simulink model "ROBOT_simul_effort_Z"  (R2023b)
settings: Solver=VariableStepAuto  StartTime=0.0  StopTime=5  RelTol=1e-3
undefined symbols (not defined in the file): deg, kg, m, manette1_Defaut_sldprt, manette2_Defaut_sldprt, mm, N, rad, s, STL, X, Y, Z
libraries: sm_lib x463, fl_lib x45, nesl_utility x27, simulink x2
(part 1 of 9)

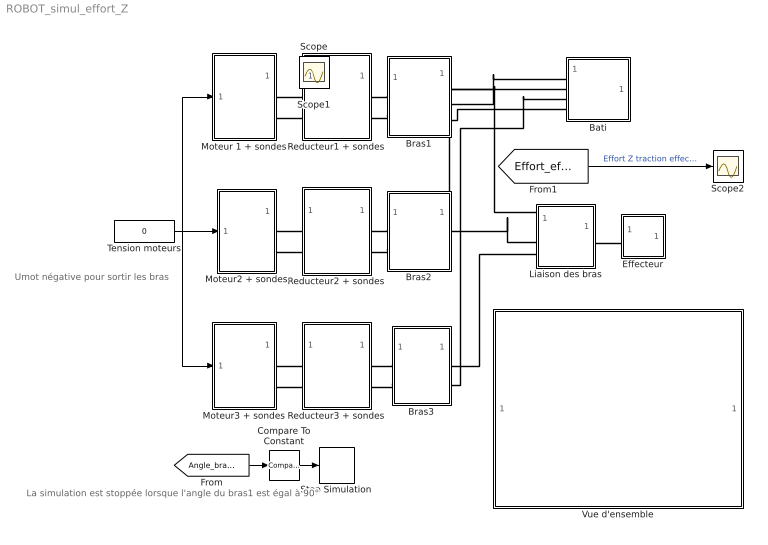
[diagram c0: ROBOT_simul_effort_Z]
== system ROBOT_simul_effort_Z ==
  note: La simulation est stoppée lorsque l'angle du bras1 est égal à 90°
  note: Umot négative pour sortir les bras
  Bati : Subsystem
  Bras1 : Subsystem
  Bras2 : Subsystem
  Bras3 : Subsystem
  Compare To Constant : simulink/Logic and Bit Operations/Compare To Constant  relop=>=  const=85  OutDataTypeStr=boolean
  Effecteur : Subsystem
  Liaison des bras : Subsystem
  Moteur 1 + sondes : Subsystem
  Moteur2 + sondes : Subsystem
  Moteur3 + sondes : Subsystem
  Reducteur1 + sondes : Subsystem
  Reducteur2 + sondes : Subsystem
  Reducteur3 + sondes : Subsystem
  Scope2 : Scope
  Stop Simulation : Stop
  Tension moteurs : Constant  Value=0
  Vue d'ensemble : Subsystem
  Scope : Scope
  Scope1 : Scope
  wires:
  [Angle_bras1] -> Compare To Constant/1
  Compare To Constant/1 -> Stop Simulation/1
  Tension moteurs/1 -> Moteur2 + sondes/1(In1), Moteur 1 + sondes/1(In1), Moteur3 + sondes/1(In1)
  [Effort_effecteur] -> Scope2/1  "Effort Z traction effecteur (N)"
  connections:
  Bras3/RConn2 -- Bati/LConn3
  Bras1/LConn2 -- Reducteur1 + sondes/RConn2
  Bras2/RConn2 -- Bati/LConn2
  Moteur3 + sondes/RConn2 -- Reducteur3 + sondes/LConn2
  Bras1/RConn2 -- Bati/LConn1
  Bras1/RConn3 -- Bati/LConn4
  Liaison des bras/LConn1 -- Bras1/RConn1
  Bras3/LConn1 -- Reducteur3 + sondes/RConn1
  Moteur 1 + sondes/RConn1 -- Reducteur1 + sondes/LConn1
  Liaison des bras/LConn3 -- Bras3/RConn1
  Liaison des bras/RConn1 -- Effecteur/LConn1
  Liaison des bras/LConn2 -- Bras2/RConn1
  Moteur2 + sondes/RConn1 -- Reducteur2 + sondes/LConn1
  Bras1/LConn1 -- Reducteur1 + sondes/RConn1
  Bras3/LConn2 -- Reducteur3 + sondes/RConn2
  Moteur2 + sondes/RConn2 -- Reducteur2 + sondes/LConn2
  Bras2/LConn2 -- Reducteur2 + sondes/RConn2
  Moteur 1 + sondes/RConn2 -- Reducteur1 + sondes/LConn2
  Bras2/LConn1 -- Reducteur2 + sondes/RConn1
  Moteur3 + sondes/RConn1 -- Reducteur3 + sondes/LConn1

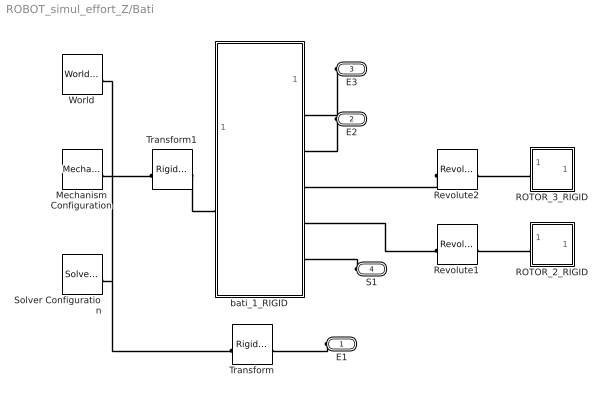
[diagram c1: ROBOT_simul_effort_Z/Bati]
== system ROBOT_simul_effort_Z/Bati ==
  Mechanism Configuration : sm_lib/Utilities/Mechanism Configuration  UniformGravity=Constant  GravityVector=[0 -9.81 0]  GravityVectorUnits=m/s^2  LinearizationDelta=0.001  JointModeTransitionNonlinearIterations=2
  ROTOR_2_RIGID : Subsystem
  ROTOR_3_RIGID : Subsystem
  Revolute1 : sm_lib/Joints/Revolute Joint  JointMode=Normal  SenseConstraintForce=off  SenseConstraintForceX=off  SenseConstraintForceY=off  SenseConstraintForceZ=off  SenseConstraintTorque=off  SenseConstraintTorqueX=off  SenseConstraintTorqueY=off  SenseConstraintTorqueZ=off  SenseTotalForce=off  SenseTotalForceX=off  SenseTotalForceY=off  SenseTotalForceZ=off  SenseTotalTorque=off  SenseTotalTorqueX=off  SenseTotalTorqueY=off  SenseTotalTorqueZ=off  CompositeWrenchDir=FollowerOnBase  CompositeWrenchFrame=BaseFrame  EquilibriumPosition=0  EquilibriumPositionUnits=rad  SpringStiffness=0  SpringStiffnessUnits=m*N/rad  DampingCoefficient=0  DampingCoefficientUnits=m*s*N/rad  TorqueActuationMode=NoTorque  MotionActuationMode=ComputedMotion  SensePosition=off  SenseVelocity=off  SenseAcceleration=off  SenseTorqueForce=off  SenseLowerLimitTorqueForce=off  SenseUpperLimitTorqueForce=off  LowerLimitSpecify=off  LowerLimitBound=-90  LowerLimitBoundUnits=deg  LowerLimitStiffness=1e4  LowerLimitStiffnessUnits=N*m/deg  LowerLimitDamping=10  LowerLimitDampingUnits=N*m/(deg/s)  LowerLimitTransitionRegionWidth=0.1  LowerLimitTransitionRegionWidthUnits=deg  UpperLimitSpecify=off  UpperLimitBound=90  UpperLimitBoundUnits=deg  UpperLimitStiffness=1e4  UpperLimitStiffnessUnits=N*m/deg  UpperLimitDamping=10  UpperLimitDampingUnits=N*m/(deg/s)  UpperLimitTransitionRegionWidth=0.1  UpperLimitTransitionRegionWidthUnits=deg  PositionTargetSpecify=on  PositionTargetPriority=Low  PositionTargetValue=-26.406351854743253  PositionTargetValueUnits=deg  VelocityTargetSpecify=off  VelocityTargetPriority=High  VelocityTargetValue=0  VelocityTargetValueUnits=deg/s
  Revolute2 : sm_lib/Joints/Revolute Joint  JointMode=Normal  SenseConstraintForce=off  SenseConstraintForceX=off  SenseConstraintForceY=off  SenseConstraintForceZ=off  SenseConstraintTorque=off  SenseConstraintTorqueX=off  SenseConstraintTorqueY=off  SenseConstraintTorqueZ=off  SenseTotalForce=off  SenseTotalForceX=off  SenseTotalForceY=off  SenseTotalForceZ=off  SenseTotalTorque=off  SenseTotalTorqueX=off  SenseTotalTorqueY=off  SenseTotalTorqueZ=off  CompositeWrenchDir=FollowerOnBase  CompositeWrenchFrame=BaseFrame  EquilibriumPosition=0  EquilibriumPositionUnits=rad  SpringStiffness=0  SpringStiffnessUnits=m*N/rad  DampingCoefficient=0  DampingCoefficientUnits=m*s*N/rad  TorqueActuationMode=NoTorque  MotionActuationMode=ComputedMotion  SensePosition=off  SenseVelocity=off  SenseAcceleration=off  SenseTorqueForce=off  SenseLowerLimitTorqueForce=off  SenseUpperLimitTorqueForce=off  LowerLimitSpecify=off  LowerLimitBound=-90  LowerLimitBoundUnits=deg  LowerLimitStiffness=1e4  LowerLimitStiffnessUnits=N*m/deg  LowerLimitDamping=10  LowerLimitDampingUnits=N*m/(deg/s)  LowerLimitTransitionRegionWidth=0.1  LowerLimitTransitionRegionWidthUnits=deg  UpperLimitSpecify=off  UpperLimitBound=90  UpperLimitBoundUnits=deg  UpperLimitStiffness=1e4  UpperLimitStiffnessUnits=N*m/deg  UpperLimitDamping=10  UpperLimitDampingUnits=N*m/(deg/s)  UpperLimitTransitionRegionWidth=0.1  UpperLimitTransitionRegionWidthUnits=deg  PositionTargetSpecify=on  PositionTargetPriority=Low  PositionTargetValue=-61.713604489421797  PositionTargetValueUnits=deg  VelocityTargetSpecify=off  VelocityTargetPriority=High  VelocityTargetValue=0  VelocityTargetValueUnits=deg/s
  Solver Configuration : nesl_utility/Solver Configuration  PhysicalDomain=network_engine_domain  SubClassName=solver  LeftPortType=input  RightPortType=generic  Tones=[]  Harmonics=[]  SimulateNoise=off  Profile=off  UseLocalSampling=off  EnableSwitchedLinearOptims=on  FrequencyDomain=off  UseCCode=off  RelTol=0.001  AbsTol=1e-06  MinStep=1e-09  ToWorkspace=off  RevertToSquareIcSolve=off  NumHomotopyIterations=100  PhasorMode=off  PhasorModeNumHarmonics=1  ConsistencySolver=NEWTON_FTOL  IndexReductionMethod=DerivativeReplacement  DoDC=off  ResidualTolerance=1e-09  ConsistencyTolSource=GLOBAL  ConsistencyAbsTol=0.001  ConsistencyRelTol=0.001  ConsistencyTolFactor=0.001  UseLocalSolver=off  LocalSolverChoice=NE_BACKWARD_EULER_ADVANCER  ResolveIndetEquations=on  FunctionEvalNumThread=1  LocalSolverSampleTime=0.001  DoFixedCost=off  MaxNonlinIter=3  MaxModeIter=2  ComputeImpulses=off  ImpulseIterations=2  LinearAlgebra=Sparse  LinearAlgebraNumThread=0  EquationFormulation=NE_TIME_EF  DelaysMemoryBudget=1024  AutomaticFiltering=on  FilteringTimeConstant=0.001  PartitionStorageMethod=AS_NEEDED  PartitionMemoryBudget=1024  PartitionMethod=FAST  MultibodyUseLocalSolver=off  MultibodyLocalSolverChoice=ODE1  MultibodyLocalSolverSampleTime=0.001
  Transform : sm_lib/Frames and Transforms/Rigid Transform  TranslationMethod=Cartesian  TranslationStandardOffset=0  TranslationStandardOffsetUnits=mm  TranslationStandardAxis=+Z  TranslationCartesianOffset=[-50.295220189469383 24.641508789034031 0]  TranslationCartesianOffsetUnits=mm  TranslationROffset=0  TranslationROffsetUnits=m  TranslationZOffset=0  TranslationZOffsetUnits=m  TranslationThetaOffset=0  TranslationThetaOffsetUnits=deg  RotationMethod=ArbitraryAxis  RotationAngleUnits=rad  RotationStandardAxis=+Z  RotationAngle=2.2576709855630148  RotationArbitraryAxis=[0.47317816576135285 0.62293756647304621 0.6229375664730461]  FollAlignAxisA=+X  BaseAlignAxisA=+Y  FollAlignAxisB=+Y  BaseAlignAxisB=+Z  RotationSequenceAxes=FollowerAxes  RotationSequence=XYX  RotationSequenceAngles=[0 0 0]  RotationSequenceAnglesUnits=deg  RotationMatrix=[1 0 0; 0 1 0; 0 0 1]  Quaternion=[1 0 0 0]
  Transform1 : sm_lib/Frames and Transforms/Rigid Transform  TranslationMethod=Cartesian  TranslationStandardOffset=0  TranslationStandardOffsetUnits=mm  TranslationStandardAxis=+Z  TranslationCartesianOffset=[0 -115.25004756062962 -99.318100969999989]  TranslationCartesianOffsetUnits=mm  TranslationROffset=0  TranslationROffsetUnits=m  TranslationZOffset=0  TranslationZOffsetUnits=m  TranslationThetaOffset=0  TranslationThetaOffsetUnits=deg  RotationMethod=None  RotationAngleUnits=deg  RotationStandardAxis=+Z  RotationAngle=0  RotationArbitraryAxis=[0 0 1]  FollAlignAxisA=+X  BaseAlignAxisA=+Y  FollAlignAxisB=+Y  BaseAlignAxisB=+Z  RotationSequenceAxes=FollowerAxes  RotationSequence=XYX  RotationSequenceAngles=[0 0 0]  RotationSequenceAnglesUnits=deg  RotationMatrix=[1 0 0; 0 1 0; 0 0 1]  Quaternion=[1 0 0 0]
  World : sm_lib/Frames and Transforms/World Frame
  bati_1_RIGID : Subsystem
  E1 : PMIOPort  Side=Left
  E2 : PMIOPort  Port=2  Side=Left
  E3 : PMIOPort  Port=3  Side=Left
  S1 : PMIOPort  Port=4  Side=Left
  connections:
  Mechanism Configuration/RConn1 -- Transform/LConn1 -- Solver Configuration/RConn1 -- World/RConn1 -- Transform1/LConn1
  ROTOR_3_RIGID/LConn1 -- Revolute2/RConn1
  Transform1/RConn1 -- bati_1_RIGID/LConn1
  Revolute2/LConn1 -- bati_1_RIGID/RConn3
  E2/RConn1 -- bati_1_RIGID/RConn2
  E1/RConn1 -- Transform/RConn1
  E3/RConn1 -- bati_1_RIGID/RConn1
  ROTOR_2_RIGID/LConn1 -- Revolute1/RConn1
  S1/RConn1 -- bati_1_RIGID/RConn5
  Revolute1/LConn1 -- bati_1_RIGID/RConn4

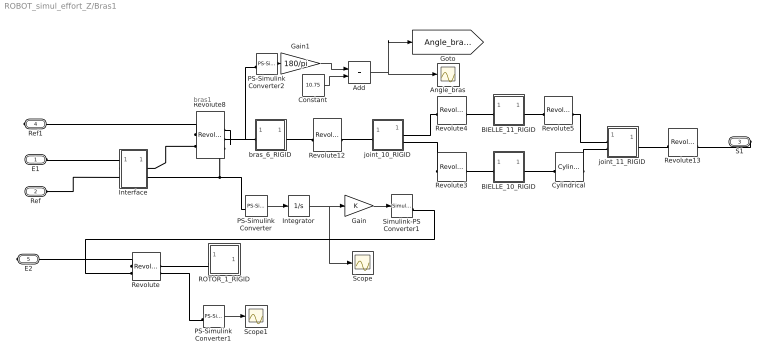
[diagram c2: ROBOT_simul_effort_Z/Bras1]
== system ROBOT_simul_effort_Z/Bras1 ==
  note: bras1
  Add : Sum
  Angle_bras : Scope
  BIELLE_10_RIGID : Subsystem
  BIELLE_11_RIGID : Subsystem
  Constant : Constant  Value=10.75
  Cylindrical : sm_lib/Joints/Cylindrical Joint  JointMode=Normal  SenseConstraintForce=off  SenseConstraintForceX=off  SenseConstraintForceY=off  SenseConstraintForceZ=off  SenseConstraintTorque=off  SenseConstraintTorqueX=off  SenseConstraintTorqueY=off  SenseConstraintTorqueZ=off  SenseTotalForce=off  SenseTotalForceX=off  SenseTotalForceY=off  SenseTotalForceZ=off  SenseTotalTorque=off  SenseTotalTorqueX=off  SenseTotalTorqueY=off  SenseTotalTorqueZ=off  CompositeWrenchDir=FollowerOnBase  CompositeWrenchFrame=BaseFrame  PzEquilibriumPosition=0  PzEquilibriumPositionUnits=m  PzSpringStiffness=0  PzSpringStiffnessUnits=N/m  PzDampingCoefficient=0  PzDampingCoefficientUnits=s*N/m  PzTorqueActuationMode=NoTorque  PzMotionActuationMode=ComputedMotion  PzSensePosition=off  PzSenseVelocity=off  PzSenseAcceleration=off  PzSenseTorqueForce=off  PzSenseLowerLimitTorqueForce=off  PzSenseUpperLimitTorqueForce=off  PzLowerLimitSpecify=off  PzLowerLimitBound=-1  PzLowerLimitBoundUnits=m  PzLowerLimitStiffness=1e6  PzLowerLimitStiffnessUnits=N/m  PzLowerLimitDamping=1e3  PzLowerLimitDampingUnits=N/(m/s)  PzLowerLimitTransitionRegionWidth=1e-4  PzLowerLimitTransitionRegionWidthUnits=m  PzUpperLimitSpecify=off  PzUpperLimitBound=1  PzUpperLimitBoundUnits=m  PzUpperLimitStiffness=1e6  PzUpperLimitStiffnessUnits=N/m  PzUpperLimitDamping=1e3  PzUpperLimitDampingUnits=N/(m/s)  PzUpperLimitTransitionRegionWidth=1e-4  PzUpperLimitTransitionRegionWidthUnits=m  PzPositionTargetSpecify=off  PzPositionTargetPriority=High  PzPositionTargetValue=0  PzPositionTargetValueUnits=m  PzVelocityTargetSpecify=off  PzVelocityTargetPriority=High  PzVelocityTargetValue=0  PzVelocityTargetValueUnits=m/s  RzEquilibriumPosition=0  RzEquilibriumPositionUnits=rad  RzSpringStiffness=0  RzSpringStiffnessUnits=m*N/rad  RzDampingCoefficient=0  RzDampingCoefficientUnits=m*s*N/rad  RzTorqueActuationMode=NoTorque  RzMotionActuationMode=ComputedMotion  RzSensePosition=off  RzSenseVelocity=off  RzSenseAcceleration=off  RzSenseTorqueForce=off  RzSenseLowerLimitTorqueForce=off  RzSenseUpperLimitTorqueForce=off  RzLowerLimitSpecify=off  RzLowerLimitBound=-90  RzLowerLimitBoundUnits=deg  RzLowerLimitStiffness=1e4  RzLowerLimitStiffnessUnits=N*m/deg  RzLowerLimitDamping=10  RzLowerLimitDampingUnits=N*m/(deg/s)  RzLowerLimitTransitionRegionWidth=0.1  RzLowerLimitTransitionRegionWidthUnits=deg  RzUpperLimitSpecify=off  RzUpperLimitBound=90  RzUpperLimitBoundUnits=deg  RzUpperLimitStiffness=1e4  RzUpperLimitStiffnessUnits=N*m/deg  RzUpperLimitDamping=10  RzUpperLimitDampingUnits=N*m/(deg/s)  RzUpperLimitTransitionRegionWidth=0.1  RzUpperLimitTransitionRegionWidthUnits=deg  RzPositionTargetSpecify=off  RzPositionTargetPriority=High  RzPositionTargetValue=0  RzPositionTargetValueUnits=deg  RzVelocityTargetSpecify=off  RzVelocityTargetPriority=High  RzVelocityTargetValue=0  RzVelocityTargetValueUnits=deg/s
  Gain : Gain
  Gain1 : Gain  Gain=180/pi
  Integrator : Integrator
  Interface : Subsystem
  PS-Simulink Converter : nesl_utility/PS-Simulink Converter  PhysicalDomain=network_engine_domain  SubClassName=ps_output  LeftPortType=input  RightPortType=output  PseudoPeriodic=off  Frequencies=[]  VectorFormat=1-D array  Unit=1  AffineConversion=off
  PS-Simulink Converter1 : nesl_utility/PS-Simulink Converter  PhysicalDomain=network_engine_domain  SubClassName=ps_output  LeftPortType=input  RightPortType=output  PseudoPeriodic=off  Frequencies=[]  VectorFormat=1-D array  Unit=1  AffineConversion=off
  PS-Simulink Converter2 : nesl_utility/PS-Simulink Converter  PhysicalDomain=network_engine_domain  SubClassName=ps_output  LeftPortType=input  RightPortType=output  PseudoPeriodic=off  Frequencies=[]  VectorFormat=1-D array  Unit=1  AffineConversion=off
  ROTOR_1_RIGID : Subsystem
  Revolute : sm_lib/Joints/Revolute Joint  JointMode=Normal  SenseConstraintForce=off  SenseConstraintForceX=off  SenseConstraintForceY=off  SenseConstraintForceZ=off  SenseConstraintTorque=off  SenseConstraintTorqueX=off  SenseConstraintTorqueY=off  SenseConstraintTorqueZ=off  SenseTotalForce=off  SenseTotalForceX=off  SenseTotalForceY=off  SenseTotalForceZ=off  SenseTotalTorque=off  SenseTotalTorqueX=off  SenseTotalTorqueY=off  SenseTotalTorqueZ=off  CompositeWrenchDir=FollowerOnBase  CompositeWrenchFrame=BaseFrame  EquilibriumPosition=0  EquilibriumPositionUnits=rad  SpringStiffness=0  SpringStiffnessUnits=m*N/rad  DampingCoefficient=0  DampingCoefficientUnits=m*s*N/rad  TorqueActuationMode=ComputedTorque  MotionActuationMode=InputMotion  SensePosition=off  SenseVelocity=on  SenseAcceleration=off  SenseTorqueForce=off  SenseLowerLimitTorqueForce=off  SenseUpperLimitTorqueForce=off  LowerLimitSpecify=off  LowerLimitBound=-90  LowerLimitBoundUnits=deg  LowerLimitStiffness=1e4  LowerLimitStiffnessUnits=N*m/deg  LowerLimitDamping=10  LowerLimitDampingUnits=N*m/(deg/s)  LowerLimitTransitionRegionWidth=0.1  LowerLimitTransitionRegionWidthUnits=deg  UpperLimitSpecify=off  UpperLimitBound=90  UpperLimitBoundUnits=deg  UpperLimitStiffness=1e4  UpperLimitStiffnessUnits=N*m/deg  UpperLimitDamping=10  UpperLimitDampingUnits=N*m/(deg/s)  UpperLimitTransitionRegionWidth=0.1  UpperLimitTransitionRegionWidthUnits=deg  PositionTargetSpecify=on  PositionTargetPriority=Low  PositionTargetValue=-79.560971310790379  PositionTargetValueUnits=deg  VelocityTargetSpecify=off  VelocityTargetPriority=High  VelocityTargetValue=0  VelocityTargetValueUnits=deg/s
  Revolute12 : sm_lib/Joints/Revolute Joint  JointMode=Normal  SenseConstraintForce=off  SenseConstraintForceX=off  SenseConstraintForceY=off  SenseConstraintForceZ=off  SenseConstraintTorque=off  SenseConstraintTorqueX=off  SenseConstraintTorqueY=off  SenseConstraintTorqueZ=off  SenseTotalForce=off  SenseTotalForceX=off  SenseTotalForceY=off  SenseTotalForceZ=off  SenseTotalTorque=off  SenseTotalTorqueX=off  SenseTotalTorqueY=off  SenseTotalTorqueZ=off  CompositeWrenchDir=FollowerOnBase  CompositeWrenchFrame=BaseFrame  EquilibriumPosition=0  EquilibriumPositionUnits=rad  SpringStiffness=0  SpringStiffnessUnits=m*N/rad  DampingCoefficient=0  DampingCoefficientUnits=m*s*N/rad  TorqueActuationMode=NoTorque  MotionActuationMode=ComputedMotion  SensePosition=off  SenseVelocity=off  SenseAcceleration=off  SenseTorqueForce=off  SenseLowerLimitTorqueForce=off  SenseUpperLimitTorqueForce=off  LowerLimitSpecify=off  LowerLimitBound=-90  LowerLimitBoundUnits=deg  LowerLimitStiffness=1e4  LowerLimitStiffnessUnits=N*m/deg  LowerLimitDamping=10  LowerLimitDampingUnits=N*m/(deg/s)  LowerLimitTransitionRegionWidth=0.1  LowerLimitTransitionRegionWidthUnits=deg  UpperLimitSpecify=off  UpperLimitBound=90  UpperLimitBoundUnits=deg  UpperLimitStiffness=1e4  UpperLimitStiffnessUnits=N*m/deg  UpperLimitDamping=10  UpperLimitDampingUnits=N*m/(deg/s)  UpperLimitTransitionRegionWidth=0.1  UpperLimitTransitionRegionWidthUnits=deg  PositionTargetSpecify=on  PositionTargetPriority=Low  PositionTargetValue=114.87234196171698  PositionTargetValueUnits=deg  VelocityTargetSpecify=off  VelocityTargetPriority=High  VelocityTargetValue=0  VelocityTargetValueUnits=deg/s
  Revolute13 : sm_lib/Joints/Revolute Joint  JointMode=Normal  SenseConstraintForce=off  SenseConstraintForceX=off  SenseConstraintForceY=off  SenseConstraintForceZ=off  SenseConstraintTorque=off  SenseConstraintTorqueX=off  SenseConstraintTorqueY=off  SenseConstraintTorqueZ=off  SenseTotalForce=off  SenseTotalForceX=off  SenseTotalForceY=off  SenseTotalForceZ=off  SenseTotalTorque=off  SenseTotalTorqueX=off  SenseTotalTorqueY=off  SenseTotalTorqueZ=off  CompositeWrenchDir=FollowerOnBase  CompositeWrenchFrame=BaseFrame  EquilibriumPosition=0  EquilibriumPositionUnits=rad  SpringStiffness=0  SpringStiffnessUnits=m*N/rad  DampingCoefficient=0  DampingCoefficientUnits=m*s*N/rad  TorqueActuationMode=NoTorque  MotionActuationMode=ComputedMotion  SensePosition=off  SenseVelocity=off  SenseAcceleration=off  SenseTorqueForce=off  SenseLowerLimitTorqueForce=off  SenseUpperLimitTorqueForce=off  LowerLimitSpecify=off  LowerLimitBound=-90  LowerLimitBoundUnits=deg  LowerLimitStiffness=1e4  LowerLimitStiffnessUnits=N*m/deg  LowerLimitDamping=10  LowerLimitDampingUnits=N*m/(deg/s)  LowerLimitTransitionRegionWidth=0.1  LowerLimitTransitionRegionWidthUnits=deg  UpperLimitSpecify=off  UpperLimitBound=90  UpperLimitBoundUnits=deg  UpperLimitStiffness=1e4  UpperLimitStiffnessUnits=N*m/deg  UpperLimitDamping=10  UpperLimitDampingUnits=N*m/(deg/s)  UpperLimitTransitionRegionWidth=0.1  UpperLimitTransitionRegionWidthUnits=deg  PositionTargetSpecify=off  PositionTargetPriority=High  PositionTargetValue=0  PositionTargetValueUnits=deg  VelocityTargetSpecify=off  VelocityTargetPriority=High  VelocityTargetValue=0  VelocityTargetValueUnits=deg/s
  Revolute3 : sm_lib/Joints/Revolute Joint  JointMode=Normal  SenseConstraintForce=off  SenseConstraintForceX=off  SenseConstraintForceY=off  SenseConstraintForceZ=off  SenseConstraintTorque=off  SenseConstraintTorqueX=off  SenseConstraintTorqueY=off  SenseConstraintTorqueZ=off  SenseTotalForce=off  SenseTotalForceX=off  SenseTotalForceY=off  SenseTotalForceZ=off  SenseTotalTorque=off  SenseTotalTorqueX=off  SenseTotalTorqueY=off  SenseTotalTorqueZ=off  CompositeWrenchDir=FollowerOnBase  CompositeWrenchFrame=BaseFrame  EquilibriumPosition=0  EquilibriumPositionUnits=rad  SpringStiffness=0  SpringStiffnessUnits=m*N/rad  DampingCoefficient=0  DampingCoefficientUnits=m*s*N/rad  TorqueActuationMode=NoTorque  MotionActuationMode=ComputedMotion  SensePosition=off  SenseVelocity=off  SenseAcceleration=off  SenseTorqueForce=off  SenseLowerLimitTorqueForce=off  SenseUpperLimitTorqueForce=off  LowerLimitSpecify=off  LowerLimitBound=-90  LowerLimitBoundUnits=deg  LowerLimitStiffness=1e4  LowerLimitStiffnessUnits=N*m/deg  LowerLimitDamping=10  LowerLimitDampingUnits=N*m/(deg/s)  LowerLimitTransitionRegionWidth=0.1  LowerLimitTransitionRegionWidthUnits=deg  UpperLimitSpecify=off  UpperLimitBound=90  UpperLimitBoundUnits=deg  UpperLimitStiffness=1e4  UpperLimitStiffnessUnits=N*m/deg  UpperLimitDamping=10  UpperLimitDampingUnits=N*m/(deg/s)  UpperLimitTransitionRegionWidth=0.1  UpperLimitTransitionRegionWidthUnits=deg  PositionTargetSpecify=on  PositionTargetPriority=Low  PositionTargetValue=-1.4448284825041595  PositionTargetValueUnits=deg  VelocityTargetSpecify=off  VelocityTargetPriority=High  VelocityTargetValue=0  VelocityTargetValueUnits=deg/s
  Revolute4 : sm_lib/Joints/Revolute Joint  JointMode=Normal  SenseConstraintForce=off  SenseConstraintForceX=off  SenseConstraintForceY=off  SenseConstraintForceZ=off  SenseConstraintTorque=off  SenseConstraintTorqueX=off  SenseConstraintTorqueY=off  SenseConstraintTorqueZ=off  SenseTotalForce=off  SenseTotalForceX=off  SenseTotalForceY=off  SenseTotalForceZ=off  SenseTotalTorque=off  SenseTotalTorqueX=off  SenseTotalTorqueY=off  SenseTotalTorqueZ=off  CompositeWrenchDir=FollowerOnBase  CompositeWrenchFrame=BaseFrame  EquilibriumPosition=0  EquilibriumPositionUnits=rad  SpringStiffness=0  SpringStiffnessUnits=m*N/rad  DampingCoefficient=0  DampingCoefficientUnits=m*s*N/rad  TorqueActuationMode=NoTorque  MotionActuationMode=ComputedMotion  SensePosition=off  SenseVelocity=off  SenseAcceleration=off  SenseTorqueForce=off  SenseLowerLimitTorqueForce=off  SenseUpperLimitTorqueForce=off  LowerLimitSpecify=off  LowerLimitBound=-90  LowerLimitBoundUnits=deg  LowerLimitStiffness=1e4  LowerLimitStiffnessUnits=N*m/deg  LowerLimitDamping=10  LowerLimitDampingUnits=N*m/(deg/s)  LowerLimitTransitionRegionWidth=0.1  LowerLimitTransitionRegionWidthUnits=deg  UpperLimitSpecify=off  UpperLimitBound=90  UpperLimitBoundUnits=deg  UpperLimitStiffness=1e4  UpperLimitStiffnessUnits=N*m/deg  UpperLimitDamping=10  UpperLimitDampingUnits=N*m/(deg/s)  UpperLimitTransitionRegionWidth=0.1  UpperLimitTransitionRegionWidthUnits=deg  PositionTargetSpecify=on  PositionTargetPriority=Low  PositionTargetValue=1.4448284825041535  PositionTargetValueUnits=deg  VelocityTargetSpecify=off  VelocityTargetPriority=High  VelocityTargetValue=0  VelocityTargetValueUnits=deg/s
  Revolute5 : sm_lib/Joints/Revolute Joint  JointMode=Normal  SenseConstraintForce=off  SenseConstraintForceX=off  SenseConstraintForceY=off  SenseConstraintForceZ=off  SenseConstraintTorque=off  SenseConstraintTorqueX=off  SenseConstraintTorqueY=off  SenseConstraintTorqueZ=off  SenseTotalForce=off  SenseTotalForceX=off  SenseTotalForceY=off  SenseTotalForceZ=off  SenseTotalTorque=off  SenseTotalTorqueX=off  SenseTotalTorqueY=off  SenseTotalTorqueZ=off  CompositeWrenchDir=FollowerOnBase  CompositeWrenchFrame=BaseFrame  EquilibriumPosition=0  EquilibriumPositionUnits=rad  SpringStiffness=0  SpringStiffnessUnits=m*N/rad  DampingCoefficient=0  DampingCoefficientUnits=m*s*N/rad  TorqueActuationMode=NoTorque  MotionActuationMode=ComputedMotion  SensePosition=off  SenseVelocity=off  SenseAcceleration=off  SenseTorqueForce=off  SenseLowerLimitTorqueForce=off  SenseUpperLimitTorqueForce=off  LowerLimitSpecify=off  LowerLimitBound=-90  LowerLimitBoundUnits=deg  LowerLimitStiffness=1e4  LowerLimitStiffnessUnits=N*m/deg  LowerLimitDamping=10  LowerLimitDampingUnits=N*m/(deg/s)  LowerLimitTransitionRegionWidth=0.1  LowerLimitTransitionRegionWidthUnits=deg  UpperLimitSpecify=off  UpperLimitBound=90  UpperLimitBoundUnits=deg  UpperLimitStiffness=1e4  UpperLimitStiffnessUnits=N*m/deg  UpperLimitDamping=10  UpperLimitDampingUnits=N*m/(deg/s)  UpperLimitTransitionRegionWidth=0.1  UpperLimitTransitionRegionWidthUnits=deg  PositionTargetSpecify=on  PositionTargetPriority=Low  PositionTargetValue=-178.55517151749589  PositionTargetValueUnits=deg  VelocityTargetSpecify=off  VelocityTargetPriority=High  VelocityTargetValue=0  VelocityTargetValueUnits=deg/s
  Revolute8 : sm_lib/Joints/Revolute Joint  JointMode=Normal  SenseConstraintForce=off  SenseConstraintForceX=off  SenseConstraintForceY=off  SenseConstraintForceZ=off  SenseConstraintTorque=off  SenseConstraintTorqueX=off  SenseConstraintTorqueY=off  SenseConstraintTorqueZ=off  SenseTotalForce=off  SenseTotalForceX=off  SenseTotalForceY=off  SenseTotalForceZ=off  SenseTotalTorque=off  SenseTotalTorqueX=off  SenseTotalTorqueY=off  SenseTotalTorqueZ=off  CompositeWrenchDir=FollowerOnBase  CompositeWrenchFrame=BaseFrame  EquilibriumPosition=0  EquilibriumPositionUnits=rad  SpringStiffness=0  SpringStiffnessUnits=m*N/rad  DampingCoefficient=0  DampingCoefficientUnits=m*s*N/rad  TorqueActuationMode=InputTorque  MotionActuationMode=ComputedMotion  SensePosition=on  SenseVelocity=on  SenseAcceleration=off  SenseTorqueForce=off  SenseLowerLimitTorqueForce=off  SenseUpperLimitTorqueForce=off  LowerLimitSpecify=off  LowerLimitBound=-90  LowerLimitBoundUnits=deg  LowerLimitStiffness=1e4  LowerLimitStiffnessUnits=N*m/deg  LowerLimitDamping=10  LowerLimitDampingUnits=N*m/(deg/s)  LowerLimitTransitionRegionWidth=0.1  LowerLimitTransitionRegionWidthUnits=deg  UpperLimitSpecify=off  UpperLimitBound=90  UpperLimitBoundUnits=deg  UpperLimitStiffness=1e4  UpperLimitStiffnessUnits=N*m/deg  UpperLimitDamping=10  UpperLimitDampingUnits=N*m/(deg/s)  UpperLimitTransitionRegionWidth=0.1  UpperLimitTransitionRegionWidthUnits=deg  PositionTargetSpecify=on  PositionTargetPriority=Low  PositionTargetValue=-11.877849818911594  PositionTargetValueUnits=deg  VelocityTargetSpecify=off  VelocityTargetPriority=High  VelocityTargetValue=0  VelocityTargetValueUnits=deg/s
  Scope : Scope
  Scope1 : Scope
  Simulink-PS Converter1 : nesl_utility/Simulink-PS Converter  PhysicalDomain=network_engine_domain  SubClassName=ps_input  LeftPortType=input  RightPortType=output  PseudoPeriodic=off  Frequencies=[]  NoiseDistribution=none  NoiseParameters=[]  Unit=1  AffineConversion=off  FilteringAndDerivatives=filter  SimscapeFilterOrder=2  InputFilterTimeConstant=1e-4  UdotUserProvided=1
  bras_6_RIGID : Subsystem
  joint_10_RIGID : Subsystem
  joint_11_RIGID : Subsystem
  E1 : PMIOPort  Side=Left
  Ref : PMIOPort  Port=2  Side=Left
  S1 : PMIOPort  Port=3  Side=Right
  Ref1 : PMIOPort  Port=4  Side=Right
  E2 : PMIOPort  Port=5  Side=Right
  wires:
  PS-Simulink Converter/1 -> Integrator/1
  Gain/1 -> Simulink-PS Converter1/1
  PS-Simulink Converter1/1 -> Scope1/1
  Integrator/1 -> Scope/1, Gain/1
  PS-Simulink Converter2/1 -> Gain1/1
  Gain1/1 -> Add/1
  Add/1 -> Angle_bras/1, [Angle_bras1]
  Constant/1 -> Add/2
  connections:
  Interface/RConn1 -- Revolute8/LConn2
  Interface/RConn2 -- Revolute8/RConn3 -- PS-Simulink Converter/LConn1
  Ref/RConn1 -- Interface/LConn2
  Interface/LConn1 -- E1/RConn1
  BIELLE_11_RIGID/LConn1 -- Revolute4/LConn1
  BIELLE_10_RIGID/RConn1 -- Cylindrical/LConn1
  Revolute4/RConn1 -- joint_10_RIGID/RConn1
  Cylindrical/RConn1 -- joint_11_RIGID/LConn2
  BIELLE_11_RIGID/RConn1 -- Revolute5/LConn1
  Revolute12/LConn1 -- bras_6_RIGID/RConn1
  Revolute12/RConn1 -- joint_10_RIGID/LConn1
  Revolute8/RConn1 -- bras_6_RIGID/LConn1
  Revolute8/LConn1 -- Ref1/RConn1
  Revolute5/RConn1 -- joint_11_RIGID/LConn1
  Revolute13/RConn1 -- joint_11_RIGID/RConn1
  S1/RConn1 -- Revolute13/LConn1
  Revolute3/RConn1 -- joint_10_RIGID/RConn2
  BIELLE_10_RIGID/LConn1 -- Revolute3/LConn1
  ROTOR_1_RIGID/LConn1 -- Revolute/RConn1
  Revolute/LConn1 -- E2/RConn1
  Revolute/LConn2 -- Simulink-PS Converter1/RConn1
  PS-Simulink Converter1/LConn1 -- Revolute/RConn2
  PS-Simulink Converter2/LConn1 -- Revolute8/RConn2

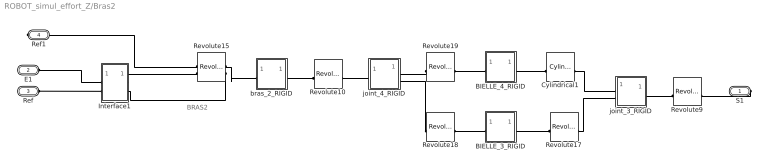
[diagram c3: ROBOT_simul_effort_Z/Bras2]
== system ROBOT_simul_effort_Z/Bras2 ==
  note: BRAS2
  BIELLE_3_RIGID : Subsystem
  BIELLE_4_RIGID : Subsystem
  Cylindrical1 : sm_lib/Joints/Cylindrical Joint  JointMode=Normal  SenseConstraintForce=off  SenseConstraintForceX=off  SenseConstraintForceY=off  SenseConstraintForceZ=off  SenseConstraintTorque=off  SenseConstraintTorqueX=off  SenseConstraintTorqueY=off  SenseConstraintTorqueZ=off  SenseTotalForce=off  SenseTotalForceX=off  SenseTotalForceY=off  SenseTotalForceZ=off  SenseTotalTorque=off  SenseTotalTorqueX=off  SenseTotalTorqueY=off  SenseTotalTorqueZ=off  CompositeWrenchDir=FollowerOnBase  CompositeWrenchFrame=BaseFrame  PzEquilibriumPosition=0  PzEquilibriumPositionUnits=m  PzSpringStiffness=0  PzSpringStiffnessUnits=N/m  PzDampingCoefficient=0  PzDampingCoefficientUnits=s*N/m  PzTorqueActuationMode=NoTorque  PzMotionActuationMode=ComputedMotion  PzSensePosition=off  PzSenseVelocity=off  PzSenseAcceleration=off  PzSenseTorqueForce=off  PzSenseLowerLimitTorqueForce=off  PzSenseUpperLimitTorqueForce=off  PzLowerLimitSpecify=off  PzLowerLimitBound=-1  PzLowerLimitBoundUnits=m  PzLowerLimitStiffness=1e6  PzLowerLimitStiffnessUnits=N/m  PzLowerLimitDamping=1e3  PzLowerLimitDampingUnits=N/(m/s)  PzLowerLimitTransitionRegionWidth=1e-4  PzLowerLimitTransitionRegionWidthUnits=m  PzUpperLimitSpecify=off  PzUpperLimitBound=1  PzUpperLimitBoundUnits=m  PzUpperLimitStiffness=1e6  PzUpperLimitStiffnessUnits=N/m  PzUpperLimitDamping=1e3  PzUpperLimitDampingUnits=N/(m/s)  PzUpperLimitTransitionRegionWidth=1e-4  PzUpperLimitTransitionRegionWidthUnits=m  PzPositionTargetSpecify=off  PzPositionTargetPriority=High  PzPositionTargetValue=0  PzPositionTargetValueUnits=m  PzVelocityTargetSpecify=off  PzVelocityTargetPriority=High  PzVelocityTargetValue=0  PzVelocityTargetValueUnits=m/s  RzEquilibriumPosition=0  RzEquilibriumPositionUnits=rad  RzSpringStiffness=0  RzSpringStiffnessUnits=m*N/rad  RzDampingCoefficient=0  RzDampingCoefficientUnits=m*s*N/rad  RzTorqueActuationMode=NoTorque  RzMotionActuationMode=ComputedMotion  RzSensePosition=off  RzSenseVelocity=off  RzSenseAcceleration=off  RzSenseTorqueForce=off  RzSenseLowerLimitTorqueForce=off  RzSenseUpperLimitTorqueForce=off  RzLowerLimitSpecify=off  RzLowerLimitBound=-90  RzLowerLimitBoundUnits=deg  RzLowerLimitStiffness=1e4  RzLowerLimitStiffnessUnits=N*m/deg  RzLowerLimitDamping=10  RzLowerLimitDampingUnits=N*m/(deg/s)  RzLowerLimitTransitionRegionWidth=0.1  RzLowerLimitTransitionRegionWidthUnits=deg  RzUpperLimitSpecify=off  RzUpperLimitBound=90  RzUpperLimitBoundUnits=deg  RzUpperLimitStiffness=1e4  RzUpperLimitStiffnessUnits=N*m/deg  RzUpperLimitDamping=10  RzUpperLimitDampingUnits=N*m/(deg/s)  RzUpperLimitTransitionRegionWidth=0.1  RzUpperLimitTransitionRegionWidthUnits=deg  RzPositionTargetSpecify=off  RzPositionTargetPriority=High  RzPositionTargetValue=0  RzPositionTargetValueUnits=deg  RzVelocityTargetSpecify=off  RzVelocityTargetPriority=High  RzVelocityTargetValue=0  RzVelocityTargetValueUnits=deg/s
  Interface1 : Subsystem
  Revolute10 : sm_lib/Joints/Revolute Joint  JointMode=Normal  SenseConstraintForce=off  SenseConstraintForceX=off  SenseConstraintForceY=off  SenseConstraintForceZ=off  SenseConstraintTorque=off  SenseConstraintTorqueX=off  SenseConstraintTorqueY=off  SenseConstraintTorqueZ=off  SenseTotalForce=off  SenseTotalForceX=off  SenseTotalForceY=off  SenseTotalForceZ=off  SenseTotalTorque=off  SenseTotalTorqueX=off  SenseTotalTorqueY=off  SenseTotalTorqueZ=off  CompositeWrenchDir=FollowerOnBase  CompositeWrenchFrame=BaseFrame  EquilibriumPosition=0  EquilibriumPositionUnits=rad  SpringStiffness=0  SpringStiffnessUnits=m*N/rad  DampingCoefficient=0  DampingCoefficientUnits=m*s*N/rad  TorqueActuationMode=NoTorque  MotionActuationMode=ComputedMotion  SensePosition=off  SenseVelocity=off  SenseAcceleration=off  SenseTorqueForce=off  SenseLowerLimitTorqueForce=off  SenseUpperLimitTorqueForce=off  LowerLimitSpecify=off  LowerLimitBound=-90  LowerLimitBoundUnits=deg  LowerLimitStiffness=1e4  LowerLimitStiffnessUnits=N*m/deg  LowerLimitDamping=10  LowerLimitDampingUnits=N*m/(deg/s)  LowerLimitTransitionRegionWidth=0.1  LowerLimitTransitionRegionWidthUnits=deg  UpperLimitSpecify=off  UpperLimitBound=90  UpperLimitBoundUnits=deg  UpperLimitStiffness=1e4  UpperLimitStiffnessUnits=N*m/deg  UpperLimitDamping=10  UpperLimitDampingUnits=N*m/(deg/s)  UpperLimitTransitionRegionWidth=0.1  UpperLimitTransitionRegionWidthUnits=deg  PositionTargetSpecify=on  PositionTargetPriority=Low  PositionTargetValue=114.872364906431  PositionTargetValueUnits=deg  VelocityTargetSpecify=off  VelocityTargetPriority=High  VelocityTargetValue=0  VelocityTargetValueUnits=deg/s
  Revolute15 : sm_lib/Joints/Revolute Joint  JointMode=Normal  SenseConstraintForce=off  SenseConstraintForceX=off  SenseConstraintForceY=off  SenseConstraintForceZ=off  SenseConstraintTorque=off  SenseConstraintTorqueX=off  SenseConstraintTorqueY=off  SenseConstraintTorqueZ=off  SenseTotalForce=off  SenseTotalForceX=off  SenseTotalForceY=off  SenseTotalForceZ=off  SenseTotalTorque=off  SenseTotalTorqueX=off  SenseTotalTorqueY=off  SenseTotalTorqueZ=off  CompositeWrenchDir=FollowerOnBase  CompositeWrenchFrame=BaseFrame  EquilibriumPosition=0  EquilibriumPositionUnits=rad  SpringStiffness=0  SpringStiffnessUnits=m*N/rad  DampingCoefficient=0  DampingCoefficientUnits=m*s*N/rad  TorqueActuationMode=InputTorque  MotionActuationMode=ComputedMotion  SensePosition=off  SenseVelocity=on  SenseAcceleration=off  SenseTorqueForce=off  SenseLowerLimitTorqueForce=off  SenseUpperLimitTorqueForce=off  LowerLimitSpecify=off  LowerLimitBound=-90  LowerLimitBoundUnits=deg  LowerLimitStiffness=1e4  LowerLimitStiffnessUnits=N*m/deg  LowerLimitDamping=10  LowerLimitDampingUnits=N*m/(deg/s)  LowerLimitTransitionRegionWidth=0.1  LowerLimitTransitionRegionWidthUnits=deg  UpperLimitSpecify=off  UpperLimitBound=90  UpperLimitBoundUnits=deg  UpperLimitStiffness=1e4  UpperLimitStiffnessUnits=N*m/deg  UpperLimitDamping=10  UpperLimitDampingUnits=N*m/(deg/s)  UpperLimitTransitionRegionWidth=0.1  UpperLimitTransitionRegionWidthUnits=deg  PositionTargetSpecify=on  PositionTargetPriority=Low  PositionTargetValue=-168.12223208512529  PositionTargetValueUnits=deg  VelocityTargetSpecify=off  VelocityTargetPriority=High  VelocityTargetValue=0  VelocityTargetValueUnits=deg/s
  Revolute17 : sm_lib/Joints/Revolute Joint  JointMode=Normal  SenseConstraintForce=off  SenseConstraintForceX=off  SenseConstraintForceY=off  SenseConstraintForceZ=off  SenseConstraintTorque=off  SenseConstraintTorqueX=off  SenseConstraintTorqueY=off  SenseConstraintTorqueZ=off  SenseTotalForce=off  SenseTotalForceX=off  SenseTotalForceY=off  SenseTotalForceZ=off  SenseTotalTorque=off  SenseTotalTorqueX=off  SenseTotalTorqueY=off  SenseTotalTorqueZ=off  CompositeWrenchDir=FollowerOnBase  CompositeWrenchFrame=BaseFrame  EquilibriumPosition=0  EquilibriumPositionUnits=rad  SpringStiffness=0  SpringStiffnessUnits=m*N/rad  DampingCoefficient=0  DampingCoefficientUnits=m*s*N/rad  TorqueActuationMode=NoTorque  MotionActuationMode=ComputedMotion  SensePosition=off  SenseVelocity=off  SenseAcceleration=off  SenseTorqueForce=off  SenseLowerLimitTorqueForce=off  SenseUpperLimitTorqueForce=off  LowerLimitSpecify=off  LowerLimitBound=-90  LowerLimitBoundUnits=deg  LowerLimitStiffness=1e4  LowerLimitStiffnessUnits=N*m/deg  LowerLimitDamping=10  LowerLimitDampingUnits=N*m/(deg/s)  LowerLimitTransitionRegionWidth=0.1  LowerLimitTransitionRegionWidthUnits=deg  UpperLimitSpecify=off  UpperLimitBound=90  UpperLimitBoundUnits=deg  UpperLimitStiffness=1e4  UpperLimitStiffnessUnits=N*m/deg  UpperLimitDamping=10  UpperLimitDampingUnits=N*m/(deg/s)  UpperLimitTransitionRegionWidth=0.1  UpperLimitTransitionRegionWidthUnits=deg  PositionTargetSpecify=on  PositionTargetPriority=Low  PositionTargetValue=-1.4448169961462776  PositionTargetValueUnits=deg  VelocityTargetSpecify=off  VelocityTargetPriority=High  VelocityTargetValue=0  VelocityTargetValueUnits=deg/s
  Revolute18 : sm_lib/Joints/Revolute Joint  JointMode=Normal  SenseConstraintForce=off  SenseConstraintForceX=off  SenseConstraintForceY=off  SenseConstraintForceZ=off  SenseConstraintTorque=off  SenseConstraintTorqueX=off  SenseConstraintTorqueY=off  SenseConstraintTorqueZ=off  SenseTotalForce=off  SenseTotalForceX=off  SenseTotalForceY=off  SenseTotalForceZ=off  SenseTotalTorque=off  SenseTotalTorqueX=off  SenseTotalTorqueY=off  SenseTotalTorqueZ=off  CompositeWrenchDir=FollowerOnBase  CompositeWrenchFrame=BaseFrame  EquilibriumPosition=0  EquilibriumPositionUnits=rad  SpringStiffness=0  SpringStiffnessUnits=m*N/rad  DampingCoefficient=0  DampingCoefficientUnits=m*s*N/rad  TorqueActuationMode=NoTorque  MotionActuationMode=ComputedMotion  SensePosition=off  SenseVelocity=off  SenseAcceleration=off  SenseTorqueForce=off  SenseLowerLimitTorqueForce=off  SenseUpperLimitTorqueForce=off  LowerLimitSpecify=off  LowerLimitBound=-90  LowerLimitBoundUnits=deg  LowerLimitStiffness=1e4  LowerLimitStiffnessUnits=N*m/deg  LowerLimitDamping=10  LowerLimitDampingUnits=N*m/(deg/s)  LowerLimitTransitionRegionWidth=0.1  LowerLimitTransitionRegionWidthUnits=deg  UpperLimitSpecify=off  UpperLimitBound=90  UpperLimitBoundUnits=deg  UpperLimitStiffness=1e4  UpperLimitStiffnessUnits=N*m/deg  UpperLimitDamping=10  UpperLimitDampingUnits=N*m/(deg/s)  UpperLimitTransitionRegionWidth=0.1  UpperLimitTransitionRegionWidthUnits=deg  PositionTargetSpecify=on  PositionTargetPriority=Low  PositionTargetValue=178.55518300385469  PositionTargetValueUnits=deg  VelocityTargetSpecify=off  VelocityTargetPriority=High  VelocityTargetValue=0  VelocityTargetValueUnits=deg/s
  Revolute19 : sm_lib/Joints/Revolute Joint  JointMode=Normal  SenseConstraintForce=off  SenseConstraintForceX=off  SenseConstraintForceY=off  SenseConstraintForceZ=off  SenseConstraintTorque=off  SenseConstraintTorqueX=off  SenseConstraintTorqueY=off  SenseConstraintTorqueZ=off  SenseTotalForce=off  SenseTotalForceX=off  SenseTotalForceY=off  SenseTotalForceZ=off  SenseTotalTorque=off  SenseTotalTorqueX=off  SenseTotalTorqueY=off  SenseTotalTorqueZ=off  CompositeWrenchDir=FollowerOnBase  CompositeWrenchFrame=BaseFrame  EquilibriumPosition=0  EquilibriumPositionUnits=rad  SpringStiffness=0  SpringStiffnessUnits=m*N/rad  DampingCoefficient=0  DampingCoefficientUnits=m*s*N/rad  TorqueActuationMode=NoTorque  MotionActuationMode=ComputedMotion  SensePosition=off  SenseVelocity=off  SenseAcceleration=off  SenseTorqueForce=off  SenseLowerLimitTorqueForce=off  SenseUpperLimitTorqueForce=off  LowerLimitSpecify=off  LowerLimitBound=-90  LowerLimitBoundUnits=deg  LowerLimitStiffness=1e4  LowerLimitStiffnessUnits=N*m/deg  LowerLimitDamping=10  LowerLimitDampingUnits=N*m/(deg/s)  LowerLimitTransitionRegionWidth=0.1  LowerLimitTransitionRegionWidthUnits=deg  UpperLimitSpecify=off  UpperLimitBound=90  UpperLimitBoundUnits=deg  UpperLimitStiffness=1e4  UpperLimitStiffnessUnits=N*m/deg  UpperLimitDamping=10  UpperLimitDampingUnits=N*m/(deg/s)  UpperLimitTransitionRegionWidth=0.1  UpperLimitTransitionRegionWidthUnits=deg  PositionTargetSpecify=on  PositionTargetPriority=Low  PositionTargetValue=-178.55518300385467  PositionTargetValueUnits=deg  VelocityTargetSpecify=off  VelocityTargetPriority=High  VelocityTargetValue=0  VelocityTargetValueUnits=deg/s
  Revolute9 : sm_lib/Joints/Revolute Joint  JointMode=Normal  SenseConstraintForce=off  SenseConstraintForceX=off  SenseConstraintForceY=off  SenseConstraintForceZ=off  SenseConstraintTorque=off  SenseConstraintTorqueX=off  SenseConstraintTorqueY=off  SenseConstraintTorqueZ=off  SenseTotalForce=off  SenseTotalForceX=off  SenseTotalForceY=off  SenseTotalForceZ=off  SenseTotalTorque=off  SenseTotalTorqueX=off  SenseTotalTorqueY=off  SenseTotalTorqueZ=off  CompositeWrenchDir=FollowerOnBase  CompositeWrenchFrame=BaseFrame  EquilibriumPosition=0  EquilibriumPositionUnits=rad  SpringStiffness=0  SpringStiffnessUnits=m*N/rad  DampingCoefficient=0  DampingCoefficientUnits=m*s*N/rad  TorqueActuationMode=NoTorque  MotionActuationMode=ComputedMotion  SensePosition=off  SenseVelocity=off  SenseAcceleration=off  SenseTorqueForce=off  SenseLowerLimitTorqueForce=off  SenseUpperLimitTorqueForce=off  LowerLimitSpecify=off  LowerLimitBound=-90  LowerLimitBoundUnits=deg  LowerLimitStiffness=1e4  LowerLimitStiffnessUnits=N*m/deg  LowerLimitDamping=10  LowerLimitDampingUnits=N*m/(deg/s)  LowerLimitTransitionRegionWidth=0.1  LowerLimitTransitionRegionWidthUnits=deg  UpperLimitSpecify=off  UpperLimitBound=90  UpperLimitBoundUnits=deg  UpperLimitStiffness=1e4  UpperLimitStiffnessUnits=N*m/deg  UpperLimitDamping=10  UpperLimitDampingUnits=N*m/(deg/s)  UpperLimitTransitionRegionWidth=0.1  UpperLimitTransitionRegionWidthUnits=deg  PositionTargetSpecify=off  PositionTargetPriority=High  PositionTargetValue=0  PositionTargetValueUnits=deg  VelocityTargetSpecify=off  VelocityTargetPriority=High  VelocityTargetValue=0  VelocityTargetValueUnits=deg/s
  bras_2_RIGID : Subsystem
  joint_3_RIGID : Subsystem
  joint_4_RIGID : Subsystem
  S1 : PMIOPort  Side=Right
  E1 : PMIOPort  Port=2  Side=Left
  Ref : PMIOPort  Port=3  Side=Left
  Ref1 : PMIOPort  Port=4  Side=Right
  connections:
  Interface1/RConn2 -- Revolute15/RConn2
  Interface1/RConn1 -- Revolute15/LConn2
  Interface1/LConn1 -- E1/RConn1
  Interface1/LConn2 -- Ref/RConn1
  BIELLE_3_RIGID/LConn1 -- Revolute17/RConn1
  Cylindrical1/LConn1 -- joint_3_RIGID/LConn1
  Revolute15/RConn1 -- bras_2_RIGID/LConn1
  Revolute10/RConn1 -- joint_4_RIGID/LConn1
  Revolute17/LConn1 -- joint_3_RIGID/LConn2
  Revolute10/LConn1 -- bras_2_RIGID/RConn1
  S1/RConn1 -- Revolute9/RConn1
  Revolute9/LConn1 -- joint_3_RIGID/RConn1
  BIELLE_3_RIGID/RConn1 -- Revolute18/LConn1
  Revolute15/LConn1 -- Ref1/RConn1
  Revolute18/RConn1 -- joint_4_RIGID/RConn2
  BIELLE_4_RIGID/LConn1 -- Cylindrical1/RConn1
  Revolute19/RConn1 -- joint_4_RIGID/RConn1
  BIELLE_4_RIGID/RConn1 -- Revolute19/LConn1
